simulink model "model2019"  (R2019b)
settings: Solver=VariableStepAuto  StartTime=0.0  StopTime=30  RelTol=1e-5
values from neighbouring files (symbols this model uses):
  A = A(1:(pocet_stavu),1:(pocet_stavu))    [appDekompLQR.m]    (also in appLQR.m = A(1:(2*N-1),1:(2*N-1)); appSYM.m = A(1:(2*N-1),1:(2*N-1)); appSZV.m = A(1:(2*N-1),1:(2*N-1)); central_LQR.m = A(1:(2*N-1),1:(2*N-1)))
  a_lead = A(1,1)    [appDekompLQR.m]    (also in distri_STRUKTURAL.m; struktural_stary.m)
  ABk1 = a1 - b1*K_lead1    [struktural_stary.m]
  ABk2 = a2 - b2*K1    [struktural_stary.m]
  B = zeros(pocet_stavu,N)    [appDekompLQR.m]    (also in appLQR.m = zeros(2*N-1,N); appSYM.m = zeros(2*N-1,N); appSZV.m = zeros(2*N-1,N); central_LQR.m = zeros(2*N-1,N))
  B1 = B(1:3,2)    [struktural_stary.m]
  B2 = B(3:5,3)    [struktural_stary.m]
  b_lead = B(1,1)    [appDekompLQR.m]    (also in distri_STRUKTURAL.m; struktural_stary.m)
  C = eye(pocet_stavu)    [appDekompLQR.m]    (also in appLQR.m; appSYM.m; appSZV.m; central_LQR.m)
  D = zeros(pocet_stavu,N)    [appDekompLQR.m]    (also in appLQR.m; appSYM.m; appSZV.m; central_LQR.m)
  K = zeros(N,pocet_stavu)    [appDekompLQR.m]    (also in appSYM.m = [[0,-1/5,0,-3/20,0,-1/10,0,-1/20,0]; appSZV.m = [[-5/2,-3,7/4,1/2,0,0,0];[-1/7,-2/7,-7/2,-37/7,18/7,0,0];[0,; central_LQR.m = -K; central_SYM.m = [[0,-1/5,0,-3/20,0,-1/10,0,-1/20,0])
undefined symbols (not defined in the file or in its folder): ABK, BC, K1, K2, K_lead, KKK
libraries: simulink x3

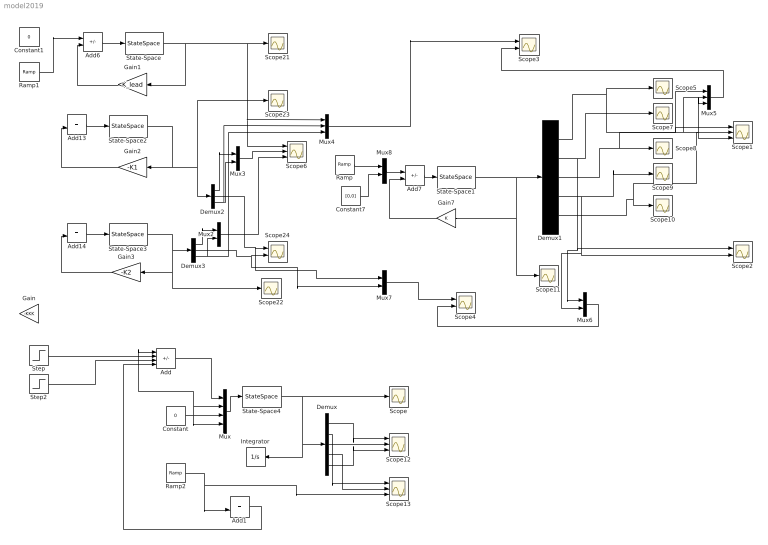
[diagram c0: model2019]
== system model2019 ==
  Add : Sum  Inputs=++-+
  Add1 : Sum
  Add13 : Sum  Commented=on
  Add14 : Sum  Commented=on
  Add6 : Sum  Commented=on  Inputs=+-
  Add7 : Sum  Commented=on  Inputs=+-
  Constant : Constant  Value=0
  Constant1 : Constant  Commented=on  Value=0
  Constant7 : Constant  Commented=on  Value=[0,0]
  Demux : Demux  Outputs=5
  Demux1 : Demux  Commented=on  Outputs=5
  Demux2 : Demux  Commented=on  Outputs=3
  Demux3 : Demux  Commented=on  Outputs=3
  Gain : Gain  Commented=on  Gain=-KKK  Multiplication=Matrix(K*u)
  Gain1 : Gain  Commented=on  Gain=K_lead
  Gain2 : Gain  Commented=on  Gain=-K1  Multiplication=Matrix(K*u)
  Gain3 : Gain  Commented=on  Gain=-K2  Multiplication=Matrix(K*u)
  Gain7 : Gain  Commented=on  Gain=K  Multiplication=Matrix(K*u)
  Integrator : Integrator
  Mux : Mux
  Mux{2..3,6..8} (5 alike) : Mux  Commented=on  Inputs=2
  Mux4 : Mux  Commented=on  Inputs=3
  Mux5 : Mux  Commented=on  Inputs=3
  Ramp : simulink/Sources/Ramp  Commented=on  slope=1  start=0  InitialOutput=0
  Ramp1 : simulink/Sources/Ramp  Commented=on  slope=1  start=0  InitialOutput=0
  Ramp2 : simulink/Sources/Ramp  slope=1  start=17  InitialOutput=0
  Scope{,5,7..11,21..23} (10 alike) : Scope
  Scope{1,6,12..13} (4 alike) : Scope  NumInputPorts=3
  Scope{2..4,24} (4 alike) : Scope  NumInputPorts=2
  State-Space : StateSpace  Commented=on  A=a_lead  B=b_lead  D=0  InitialCondition=1
  State-Space1 : StateSpace  Commented=on  A=A  B=B  C=C  D=D  InitialCondition=[0 1 0 0 0]
  State-Space2 : StateSpace  Commented=on  A=ABk1  B=B1  C=eye(3)  D=zeros(3,1)  InitialCondition=[0 0 0]
  State-Space3 : StateSpace  Commented=on  A=ABk2  B=B2  C=eye(3)  D=zeros(3,1)  InitialCondition=[0 0 0]
  State-Space4 : StateSpace  A=ABK  B=BC  C=eye(5)  D=zeros(5,4)  InitialCondition=[0 , -4.3 , 0 , 2.1 , 2.5]
  Step : Step  Time=10  After=2  SampleTime=0
  Step2 : Step  Time=11  After=2  SampleTime=0
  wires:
  Demux1/1 -> Mux5/1, Scope1/1, Scope5/1
  Demux1/2 -> Scope2/1, Mux6/1, Scope7/1
  Demux1/4 -> Scope2/2, Mux6/2, Scope9/1
  State-Space1/1 -> Gain7/1, Scope11/1, Demux1/1
  Demux1/5 -> Mux5/3, Scope1/3, Scope10/1
  Demux1/3 -> Mux5/2, Scope1/2, Scope8/1
  State-Space/1 -> Gain1/1, Mux4/1, Scope6/1, Scope21/1
  Add6/1 -> State-Space/1
  Gain7/1 -> Add7/2
  Add7/1 -> State-Space1/1
  Gain1/1 -> Add6/2
  State-Space2/1 -> Gain2/1, Scope23/1, Demux2/1
  State-Space3/1 -> Gain3/1, Scope22/1, Demux3/1
  Demux3/2 -> Mux7/2, Scope24/2
  Demux2/2 -> Mux7/1, Scope24/1
  Demux3/1 -> Mux2/1
  Demux3/3 -> Mux4/3, Mux2/2
  Mux2/1 -> Scope6/3
  Demux2/3 -> Mux4/2, Mux3/2
  Demux2/1 -> Mux3/1
  Mux3/1 -> Scope6/2
  Gain2/1 -> Add13/2
  Mux4/1 -> Scope3/1
  Mux5/1 -> Scope3/2
  Mux6/1 -> Scope4/2
  Mux7/1 -> Scope4/1
  Constant7/1 -> Mux8/2
  Mux8/1 -> Add7/1
  Ramp/1 -> Mux8/1
  Ramp1/1 -> Add6/1
  Add13/1 -> State-Space2/1
  Add14/1 -> State-Space3/1
  Gain3/1 -> Add14/2
  State-Space4/1 -> Demux/1, Integrator/1, Scope/1
  Demux/1 -> Scope12/1
  Demux/3 -> Scope12/2
  Demux/5 -> Scope12/3
  Demux/2 -> Scope13/1
  Demux/4 -> Scope13/2
  Step/1 -> Add/2
  Mux/1 -> State-Space4/1
  Constant/1 -> Mux/3, Mux/4, Add/1, Mux/2
  Ramp2/1 -> Scope13/3, Add1/2
  Step2/1 -> Add/3
  Add1/1 -> Add/4
  Add/1 -> Mux/1
